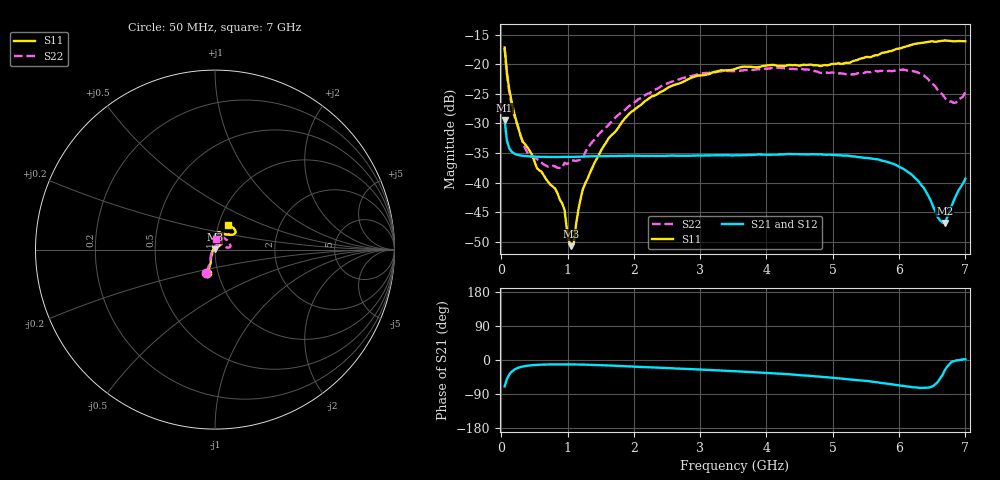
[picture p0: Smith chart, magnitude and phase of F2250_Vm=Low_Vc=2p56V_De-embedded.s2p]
! Integrated Device Technology
! Corporate Headquarters
! 6024 Silver Creek Valley Road
! San Jose, CA 95138  USA
! Phone:  1-408-284-8200
! Toll Free:  1-800-223-1366
! Webpage:  http://www.idt.com/
! Timing and RF Division
! 515 Groton Road, Suite 102
! Westford, MA 01886-6024
! Device:  F2250
! Description: Voltage Variable RF Attenuator
! Frequency:  50.0 -  6000.00 MHz
! Package:  3x3 mm Thin QFN Plastic Package: 16 pin
! Ports:  2 RF, 3 DC
!  Pin  1  = GND
!  Pin  2  = NC
!  Pin  3  = RF1  = Port 1
!  Pin  4  = NC
!  Pin  5  = GND
!  Pin  6  = GND
!  Pin  7  = GND
!  Pin  8  = GND
!  Pin  9  = NC
!  Pin 10  = RF2  = Port 2
!  Pin 11  = NC
!  Pin 12  = GND
!  Pin 13  = GND
!  Pin 14  = VCNTRL
!  Pin 15  = VDD
!  Pin 16  = VMODE
! Vcntrl:  2.560 Volts
! Vmode:  +0.000 Volts
! Vdd:  +3.30  Volts
! Current:  1.176 mA
! Data:  The device was measured on a the F2250 evaluation board which has
!  individual transmission lines to the RF pins.  Data was collected
!  using a calibrated network analyzer.  The evaluation board was
!  de-embedded using a TRL calibration technique.
!  The reference plane is the edge of the package pin.
! Misc:  SN 10
!  Action Tracker AT0258
! Date Measured:  2014-11-26
! Date:  2015-10-15  MJV
! Note:
!  Integrated Device Technology supplies this data as a sample of measured
!  data at the package pin for this product.  Your particular data for this
!  product may vary.
!  Data was taken at 25 degrees C.
!  Integrated Device Technology reserves the right to change this data at anytime.
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# GHz S dB R 50
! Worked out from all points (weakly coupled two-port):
!   201 points, 50 MHz to 7 GHz, reference 50 ohm
!   highest |S21| = -29.41 dB at 50 MHz (marker M1); lowest = -46.8 dB at 6.687 GHz (marker M2)
!   lowest |S11| = -50.8 dB at 1.058 GHz (marker M3), VSWR 1.01, Z = 49.8 + j0.241 ohm
!   |S11| at or under -10 dB: start of sweep to end of sweep
!   |S22| runs from -37.5 to -17.3 dB; largest |S21 - S12| = 6.5e-05
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0.05  -17.18 -108.6  -29.41 -69.8  -29.41 -69.8  -17.28 -111.0
0.08475  -21.45 -107.4  -32.92 -50.4  -32.92 -50.3  -21.75 -110.2
0.15425  -26.23 -116.6  -34.76 -31.1  -34.75 -31.1  -26.81 -122.4
0.29325  -32.20 -127.7  -35.44 -18.5  -35.43 -18.4  -32.10 -137.5
0.3975  -34.09 -141.8  -35.56 -15.0  -35.56 -15.0  -35.03 -160.4
0.91875  -43.52 157.8  -35.69 -11.5  -35.68 -11.5  -37.53 133.5
0.9535  -44.61 170.1  -35.69 -11.5  -35.68 -11.5  -36.67 131.3
1.023  -50.00 143.8  -35.67 -11.6  -35.67 -11.6  -36.61 116.0
1.05775  -50.75 123.5  -35.67 -11.6  -35.66 -11.6  -36.31 110.7
1.0925  -50.35 89.6  -35.66 -11.7  -35.66 -11.7  -36.29 106.2
1.162  -44.62 57.1  -35.64 -11.9  -35.64 -11.9  -36.23 95.5
1.2315  -41.10 44.3  -35.61 -12.1  -35.61 -12.1  -35.79 85.9
1.61375  -32.59 40.9  -35.52 -14.5  -35.53 -14.4  -30.30 65.6
1.9265  -28.40 41.3  -35.47 -16.9  -35.46 -16.9  -27.09 56.7
2.37825  -24.87 47.4  -35.48 -20.3  -35.48 -20.3  -23.99 56.9
3.525  -20.80 72.5  -35.41 -29.5  -35.41 -29.5  -21.19 74.8
4.7065  -20.17 72.3  -35.20 -42.5  -35.20 -42.6  -21.14 72.3
5.85325  -17.81 40.5  -36.64 -63.2  -36.63 -63.3  -21.13 23.0
6.27025  -16.50 40.1  -39.50 -72.5  -39.51 -72.7  -21.36 9.7
6.68725  -15.99 48.8  -46.85 -27.7  -46.84 -27.3  -25.64 28.5
6.861  -16.13 55.1  -42.18 -1.3  -42.13 -1.3  -26.46 57.9
7  -16.12 63.2  -39.35 1.9  -39.30 1.7  -24.63 83.1
